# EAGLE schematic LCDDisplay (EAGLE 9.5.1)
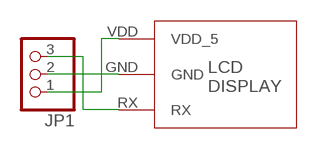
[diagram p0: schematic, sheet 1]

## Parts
JP1  PINHD-1X3  [1X03]
U$1  ADAFRUIT-782  [LCD-3]

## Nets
GND: JP1.2 U$1.GND
N$3: JP1.3 U$1.RX
VDD_5: JP1.1 U$1.VDD(VDD_5)

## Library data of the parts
JP1 = pinhead:PINHD-1X3: PIN HEADER
U$1 = MILESTONE4LIB_E:ADAFRUIT-782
